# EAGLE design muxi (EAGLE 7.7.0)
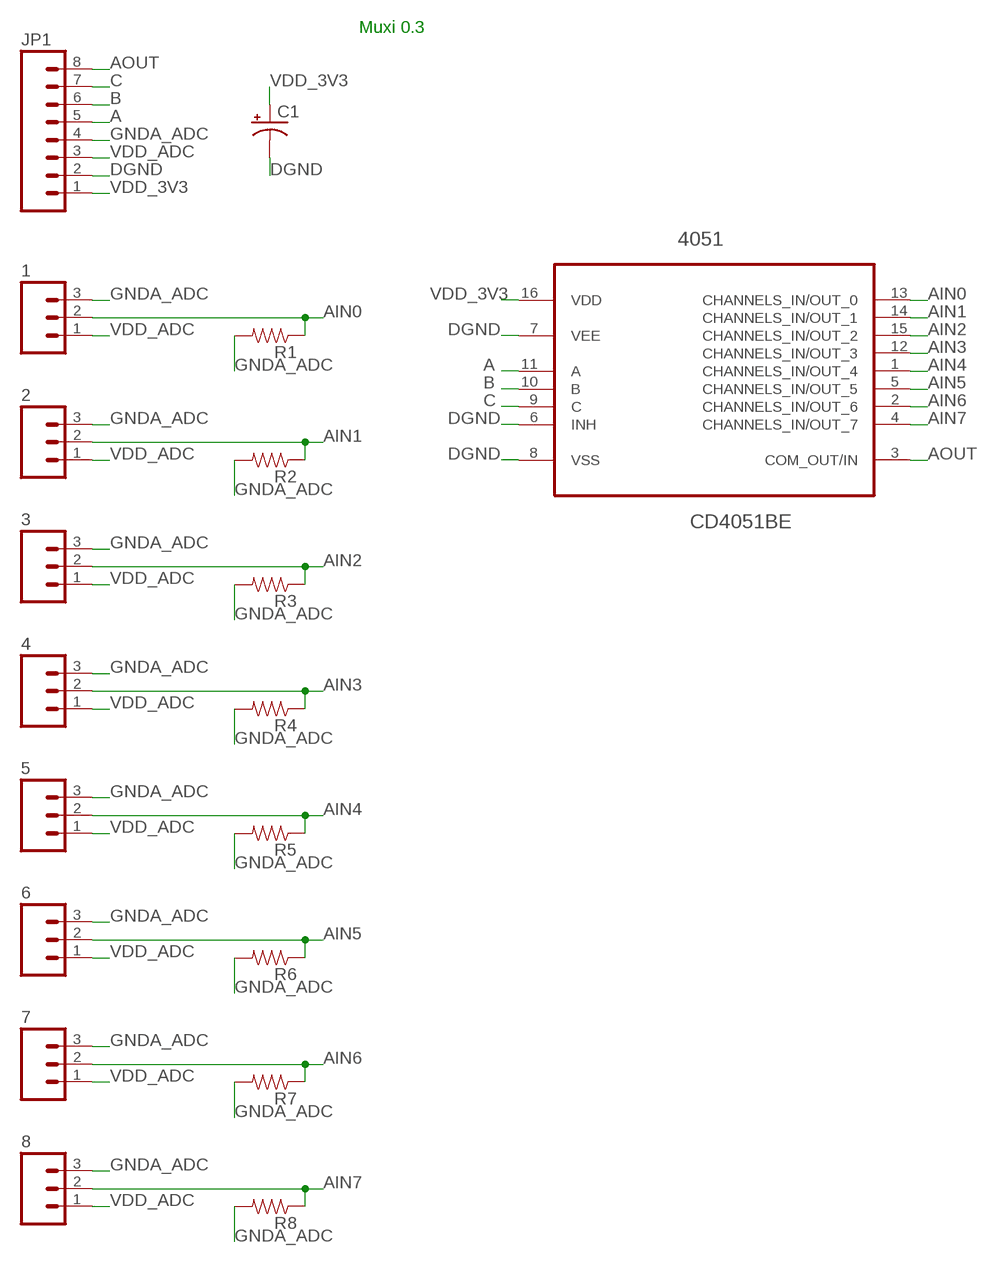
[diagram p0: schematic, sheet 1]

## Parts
1  M03PTH  [1X03]
2  M03PTH  [1X03]
3  M03PTH  [1X03]
4  M03PTH  [1X03]
5  M03PTH  [1X03]
6  M03PTH  [1X03]
7  M03PTH  [1X03]
8  M03PTH  [1X03]
4051  CD4051BE  [DIP254P762X508-16]
C1  CAP_POLPTH2  [CPOL-RADIAL-10UF-25V]
JP1  M08  [1X08_PIN1_NO_SILK]
R1  RESISTORAXIAL-0.3  [AXIAL-0.3]
R2  RESISTORAXIAL-0.3  [AXIAL-0.3]
R3  RESISTORAXIAL-0.3  [AXIAL-0.3]
R4  RESISTORAXIAL-0.3  [AXIAL-0.3]
R5  RESISTORAXIAL-0.3  [AXIAL-0.3]
R6  RESISTORAXIAL-0.3  [AXIAL-0.3]
R7  RESISTORAXIAL-0.3  [AXIAL-0.3]
R8  RESISTORAXIAL-0.3  [AXIAL-0.3]

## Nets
A: 4051.11(A) JP1.5
AIN0: 1.2 4051.13(CHANNELS_IN/OUT_0) R1.P$1
AIN1: 2.2 4051.14(CHANNELS_IN/OUT_1) R2.P$1
AIN2: 3.2 4051.15(CHANNELS_IN/OUT_2) R3.P$1
AIN3: 4.2 4051.12(CHANNELS_IN/OUT_3) R4.P$1
AIN4: 5.2 4051.1(CHANNELS_IN/OUT_4) R5.P$1
AIN5: 6.2 4051.5(CHANNELS_IN/OUT_5) R6.P$1
AIN6: 7.2 4051.2(CHANNELS_IN/OUT_6) R7.P$1
AIN7: 8.2 4051.4(CHANNELS_IN/OUT_7) R8.P$1
AOUT: 4051.3(COM_OUT/IN) JP1.8
B: 4051.10(B) JP1.6
C: 4051.9(C) JP1.7
DGND: 4051.6(INH) 4051.7(VEE) 4051.8(VSS) C1.2(-) JP1.2
GNDA_ADC: 1.3 2.3 3.3 4.3 5.3 6.3 7.3 8.3 JP1.4 R1.P$2 R2.P$2 R3.P$2 R4.P$2 R5.P$2 R6.P$2 R7.P$2 R8.P$2
VDD_3V3: 4051.16(VDD) C1.1(+) JP1.1
VDD_ADC: 1.1 2.1 3.1 4.1 5.1 6.1 7.1 8.1 JP1.3

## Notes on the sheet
- Muxi 0.3

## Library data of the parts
1-8 = SparkFun-Connectors:M03: Header 3 Standard 3-pin 0.1" header. Use with straight break away headers (SKU : PRT-00116), right angle break away headers (PRT-00553), swiss pins (PRT-00743), machine pins (PRT-00117), and female headers (PRT-00115). Molex polarized connector foot print use with SKU : PRT-08232 with associated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
4051 = my4051:CD4051BE: The CD4051B is a single 8-Channel multiplexer having three binary control inputs.; MPN: CD4051BE; OC_FARNELL: 2135100; OC_NEWARK: 60K5119; PACKAGE: PDIP-16; SUPPLIER: Texas Instruments
C1 = SparkFun-Capacitors:CAP_POL: Capacitor Polarized
JP1 = SparkFun-Connectors:M08: Header 8 Standard 8-pin 0.1" header. Use with straight break away headers (SKU : PRT-00116), right angle break away headers (PRT-00553), swiss pins (PRT-00743), machine pins (PRT-00117), and female headers (PRT-00115).
R1-R8 = SparkFun-Resistors:RESISTOR: Resistor

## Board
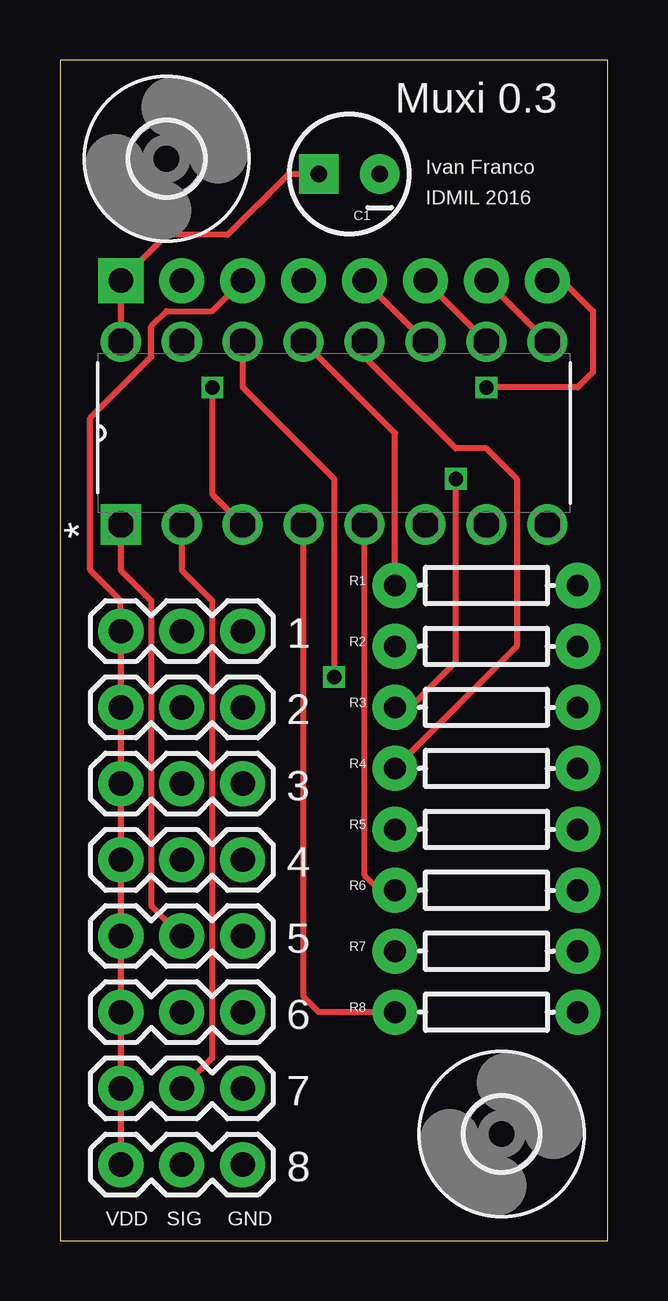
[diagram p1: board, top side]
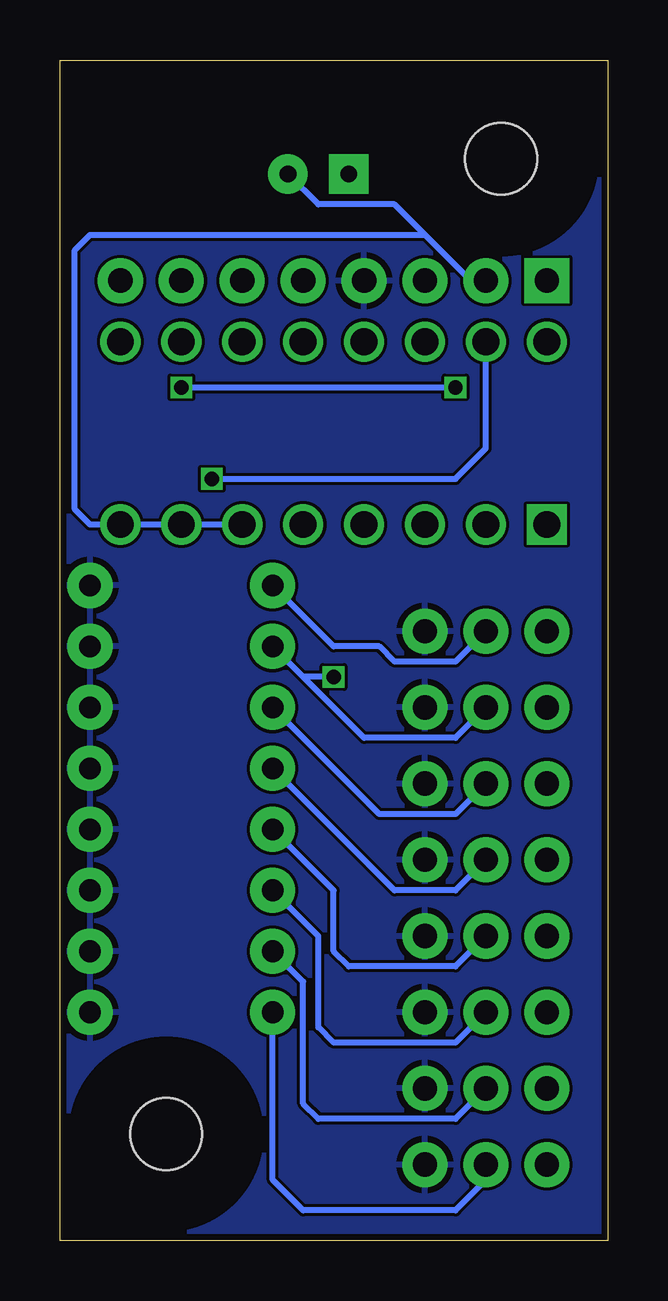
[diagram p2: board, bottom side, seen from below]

Size 22.84 x 49.2 mm. Coordinates in mm from the lower left corner, seen from the top.
Outline: 0,0 22.84,0 22.84,49.2 0,49.2 0,0
Copper layers (1*16): Top 0.035mm / dielectric 1.5mm / Bottom 0.035mm
Design rules "dirt_cheap_dirty_boards.v1": minimum track width 5mil, minimum drill 12mil, track to track 5mil, track to pad 5mil, pad to pad 5mil, via to via 5mil, smd to smd 0mil, copper to edge 10mil, drill to drill 10mil, minimum pad ring 10mil, minimum via ring 6mil, stop-mask expansion 2mil, vias tented up to drill 25mil, thermal gap 10mil

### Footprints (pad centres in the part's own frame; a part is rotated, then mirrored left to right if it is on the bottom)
1X03 = drill 1.016 pad 1.88: 1 0,0; 2 2.54,0; 3 5.08,0
DIP254P762X508-16 = drill 1.118 square: 1 -7.62,17.78 | drill 1.118: 2 -7.62,15.24; 3 -7.62,12.7; 4 -7.62,10.16; 5 -7.62,7.62; 6 -7.62,5.08; 7 -7.62,2.54; 8 -7.62,0; 9 0,0; 10 0,2.54; 11 0,5.08; 12 0,7.62; 13 0,10.16; 14 0,12.7; 15 0,15.24; 16 0,17.78
CPOL-RADIAL-10UF-25V = drill 0.7 pad 1.651 square: 1 1.27,0 | drill 0.7 pad 1.651: 2 -1.27,0
1X08_PIN1_NO_SILK = drill 1.016 pad 1.88 square: 1 0,0 | drill 1.016 pad 1.88: 2 2.54,0; 3 5.08,0; 4 7.62,0; 5 10.16,0; 6 12.7,0; 7 15.24,0; 8 17.78,0
AXIAL-0.3 = drill 0.9 pad 1.88: P$1 -3.81,0; P$2 3.81,0
3,0 = hole 3: 0,0

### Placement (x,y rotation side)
1  2.54,25.4 0 top
2  2.54,22.23 0 top
3  2.54,19.05 0 top
4  2.54,15.88 0 top
5  2.54,12.7 0 top
6  2.54,9.53 0 top
7  2.54,6.35 0 top
8  2.54,3.17 0 top
4051  20.32,37.47 90 top
C1  12.06,44.45 180 top
JP1  2.54,40.01 0 top
R1  17.78,27.3 0 top
R2  17.78,24.77 0 top
R3  17.78,22.23 0 top
R4  17.78,19.68 0 top
R5  17.78,17.14 0 top
R6  17.78,14.61 0 top
R7  17.78,12.06 0 top
R8  17.78,9.53 0 top
U$1  [3,0]  4.45,45.09 0 top
U$2  [3,0]  18.41,4.45 0 top

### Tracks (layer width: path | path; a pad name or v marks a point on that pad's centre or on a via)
A
  Top 0.254: JP1.5 4051.11
AIN0
  Top 0.254: R1.P$1 13.97,33.66 4051.13
  Bottom 0.254: 1.2 6.35,24.13 8.89,24.13 9.53,24.77 11.43,24.77 R1.P$1
AIN1  (via drill 0.6)
  Top 0.254: 4051.14 7.62,35.56 11.43,31.75 v11.43,23.5
  Bottom 0.254: 2.2 6.35,20.95 10.16,20.95 R2.P$1 12.7,23.5 v11.43,23.5
AIN2  (via drill 0.6)
  Top 0.254: R3.P$1 14.61,22.23 16.51,24.13 v16.51,31.75
  Bottom 0.254: 3.2 6.35,17.78 9.53,17.78 R3.P$1 | v16.51,31.75 6.35,31.75 5.08,33.02 4051.15
AIN3
  Top 0.254: 4051.12 12.7,36.83 16.51,33.02 17.78,33.02 19.05,31.75 19.05,24.77 R4.P$1
  Bottom 0.254: 4.2 6.35,14.61 8.89,14.61 R4.P$1
AIN4
  Top 0.254: 4051.1 2.54,27.94 3.81,26.67 3.81,13.97 5.2
  Bottom 0.254: 5.2 6.35,11.43 10.79,11.43 11.43,12.06 11.43,14.61 R5.P$1
AIN5
  Top 0.254: R6.P$1 13.34,14.61 12.7,15.24 4051.5
  Bottom 0.254: 6.2 6.35,8.26 11.43,8.26 12.06,8.89 12.06,12.7 R6.P$1
AIN6
  Top 0.254: 4051.2 5.08,27.94 6.35,26.67 6.35,7.62 7.2
  Bottom 0.254: 7.2 6.35,5.08 12.06,5.08 12.7,5.71 12.7,10.79 R7.P$1
AIN7
  Top 0.254: R8.P$1 10.79,9.53 10.16,10.16 4051.4
  Bottom 0.254: 8.2 5.08,2.54 6.35,1.27 12.7,1.27 13.97,2.54 R8.P$1
AOUT  (via drill 0.6)
  Top 0.254: JP1.8 20.95,40.01 22.23,38.73 22.23,36.2 21.59,35.56 v17.78,35.56 | v6.35,35.56 6.35,31.11 4051.3
  Bottom 0.254: v17.78,35.56 v6.35,35.56
B
  Top 0.254: JP1.6 4051.10
C
  Top 0.254: JP1.7 4051.9
DGND
  Bottom 0.254: JP1.2 5.71,40.01 7.62,41.91 | 7.62,41.91 8.89,43.18 12.06,43.18 C1.2 | 4051.8 4051.7 4051.6 21.59,29.84 22.23,30.48 22.23,41.27 21.59,41.91 7.62,41.91
GNDA_ADC
  pour Bottom: 0,49.53 22.86,49.53 22.86,0 0,0
VDD_3V3
  Top 0.254: C1.1 9.53,44.45 6.99,41.91 4.45,41.91 JP1.1 4051.16
VDD_ADC
  Top 0.254: 8.1 7.1 6.1 5.1 4.1 3.1 2.1 1.1 2.54,26.67 1.27,27.94 1.27,34.29 3.81,36.83 3.81,38.1 4.45,38.73 6.35,38.73 JP1.3

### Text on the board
tNames: Muxi 0.3 | Ivan Franco | IDMIL 2016 | VDD | SIG | GND

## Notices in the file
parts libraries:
SparkFun-Connectors: Licensing: Creative Commons ShareAlike 4.0 International - https://creativecommons.org/licenses/by-sa/4.0
